ORGANIZATION_BLOCK MAIN:OB1
TITLE=

BEGIN
NETWORK 1
LD SM0.1
R M0.2 1
R M0.1 1


NETWORK 2
LD I0.2
A I0.3
= M1.1

NETWORK 3
LDN I0.2
AN I0.3
= M1.0

NETWORK 4
LD I0.0
LD M1.0
CTU C1 +60

NETWORK 5
LD I0.1
LD M1.0
CTU C2 +100

NETWORK 6
LD I0.6
O M0.2
A I0.7
= M0.2

NETWORK 7
LD M0.2
AN C1
AN M1.1
= Q0.1
= Q0.0


NETWORK 8
LD M0.2
AN C2
AN M1.1
= Q0.2
= Q0.3


NETWORK 9
LD C1
A C2
O M1.1
EU
S M0.1 1

NETWORK 10
LD M0.2
A M0.1
TON T32 +200

NETWORK 11
LD M0.2
AN Q0.4
A M0.1
= Q0.5
= Q1.6


NETWORK 12
LD T32
EU
S M2.0 1
R M0.1 1


NETWORK 13
LD M2.0
O Q0.4
A M0.2
AN M1.0
= Q0.4

NETWORK 14
LD M1.0
EU
R M2.0 1

NETWORK 15
LD Q0.1
= Q0.6

NETWORK 16
LD Q0.2
= Q0.7

NETWORK 17
LD Q0.5
= Q1.0

NETWORK 18
LD Q0.4
= Q1.1

END_ORGANIZATION_BLOCK

